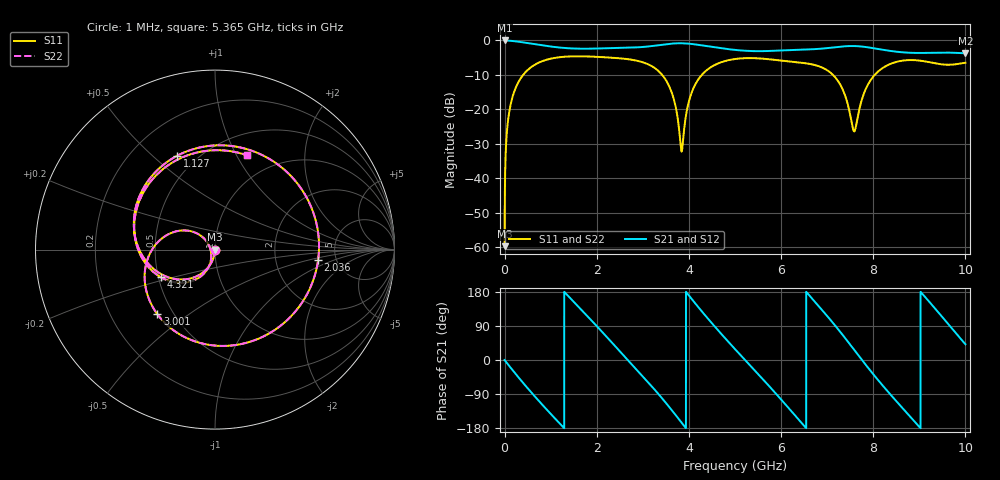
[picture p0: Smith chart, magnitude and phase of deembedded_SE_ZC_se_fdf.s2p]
# GHz S MA R 50
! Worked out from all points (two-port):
!   10000 points, 1 MHz to 10 GHz, reference 50 ohm
!   highest |S21| = 0.00 dB at 1 MHz (marker M1); lowest = -3.7 dB at 10 GHz (marker M2)
!   |S21| within 3 dB of the highest: start of sweep to 5.242 GHz; 5.834 GHz to 8.353 GHz (2.52 GHz wide, 35.5 % of centre)
!   lowest |S11| = -59.6 dB at 1 MHz (marker M3), VSWR 1.00, Z = 50 - j0.104 ohm
!   |S11| at or under -10 dB: start of sweep to 402.5 MHz; 3.42 GHz to 4.279 GHz (858.8 MHz wide, 22.3 % of centre); 7.127 GHz to 8.031 GHz (904.2 MHz wide, 11.9 % of centre)
!   |S22| runs from -59.6 to -4.6 dB; largest |S21 - S12| = 1.4e-15
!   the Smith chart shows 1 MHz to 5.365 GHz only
!   S11 on the Smith chart (normalised r, x): 1 MHz: 1.00, -0.00; 1.127 GHz: 0.39, +0.60; 2.036 GHz: 3.61, -0.63; 3.001 GHz: 0.41, -0.38; 4.321 GHz: 0.52, -0.18; 5.365 GHz: 0.73, +1.10
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0.001  0.001045 -94.1  0.9999 -0.2  0.9999 -0.2  0.001045 -94.1
0.07  0.06465 -103.7  0.9951 -10.9  0.9951 -10.9  0.06465 -103.7
0.215  0.1856 -125.5  0.9754 -32.9  0.9754 -32.9  0.1856 -125.5
0.621  0.4298 177.7  0.8895 -91.2  0.8895 -91.2  0.4298 177.7
1.127  0.5638 112.0  0.798 -158.5  0.798 -158.5  0.5638 112.0
1.668  0.589 42.3  0.7594 132.5  0.7594 132.5  0.589 42.3
2.036  0.5775 -5.8  0.765 84.9  0.765 84.9  0.5775 -5.8
2.552  0.547 -73.1  0.78 16.3  0.78 16.3  0.547 -73.1
3.001  0.4825 -131.7  0.8043 -43.4  0.8043 -43.4  0.4825 -131.7
3.334  0.3631 -176.7  0.8528 -89.0  0.8528 -89.0  0.3631 -176.7
3.842  0.02451 -166.9  0.9101 -165.4  0.9101 -165.4  0.02451 -166.9
4.321  0.3386 -152.9  0.8407 122.4  0.8407 122.4  0.3386 -152.9
5.001  0.5383 118.3  0.7292 28.7  0.7292 28.7  0.5383 118.3
5.365  0.5548 71.2  0.7019 -19.2  0.7019 -19.2  0.5548 71.2
5.994  0.5116 -13.3  0.7158 -103.2  0.7158 -103.2  0.5116 -13.3
6.667  0.451 -104.7  0.7445 163.1  0.7445 163.1  0.451 -104.7
7.208  0.2741 -176.2  0.8021 85.8  0.8021 85.8  0.2741 -176.2
7.669  0.08131 -113.8  0.8249 13.7  0.8249 13.7  0.08131 -113.8
8.334  0.445 179.4  0.711 -85.6  0.711 -85.6  0.445 179.4
9.096  0.5008 82.3  0.6596 170.4  0.6596 170.4  0.5008 82.3
9.57  0.4452 12.9  0.667 103.1  0.667 103.1  0.4452 12.9
10  0.4756 -50.4  0.6515 41.6  0.6515 41.6  0.4756 -50.4
